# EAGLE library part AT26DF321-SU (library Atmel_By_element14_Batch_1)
Serial Firmware Data Flash Memory
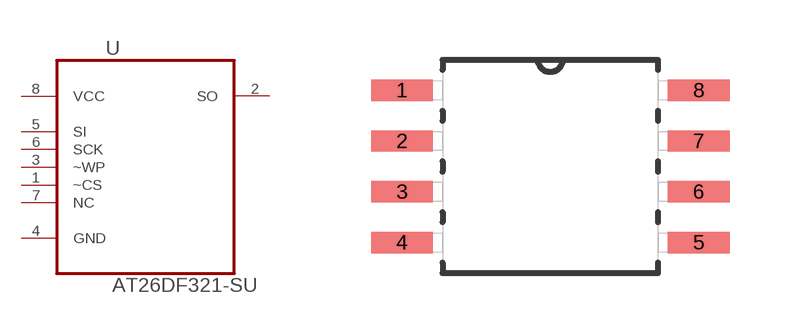
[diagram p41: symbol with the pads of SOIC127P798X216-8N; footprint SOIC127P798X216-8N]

Designator prefix U

## AT26DF321-SU (MPN: AT26DF321-SU; OC_FARNELL: 1455017; OC_NEWARK: 58M3816; PACKAGE: SOIC-8; SUPPLIER: Atmel)  [SOIC127P798X216-8N]
1  ~CS  in
2  SO  out
3  ~WP  in
4  GND  pas
5  SI  in
6  SCK  in
7  NC  nc
8  VCC  pwr

## Footprint SOIC127P798X216-8N (pad centres in mm)
smd 1.549 x 0.533: 1 -3.708,1.905; 2 -3.708,0.635; 3 -3.708,-0.635; 4 -3.708,-1.905; 5 3.708,-1.905; 6 3.708,-0.635; 7 3.708,0.635; 8 3.708,1.905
